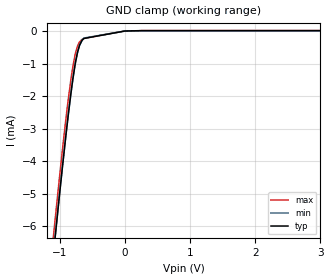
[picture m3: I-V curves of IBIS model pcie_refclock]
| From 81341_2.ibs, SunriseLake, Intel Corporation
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[Model]   pcie_refclock
Model_type   Input
Vinl = 120mV
Vinh = 1000mV
|   typ   min   max
C_comp   600.000fF   500.000fF   700.000fF
[Voltage Range]   1.800V   1.710V   1.890V
[Temperature Range]   60.0   105.0   0.0
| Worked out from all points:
|   GND clamp passes 1 mA (typ) near -0.76 V on its own axis
[GND Clamp]
|   Voltage   I(typ)   I(min)   I(max)
-1.8V     -21.74mA   -21.55mA   -21.76mA
-1.11V    -7.061mA   -7.048mA   -6.513mA
-1.08V    -6.464mA   -6.454mA   -5.917mA
-1.01V    -5.097mA   -5.093mA   -4.558mA
-910mV    -3.236mA   -3.24mA    -2.733mA
-870mV    -2.541mA   -2.549mA   -2.069mA
-800mV    -1.453mA   -1.465mA   -1.079mA
-730mV    -656.1uA   -662.6uA   -463.7uA
-700mV    -445.8uA   -446.4uA   -337.5uA
-630mV    -229.4uA   -216.1uA   -226uA
0V        60.95pA    29.85pA    35.43pA
3.6V      10.65uA    8.798uA    13.22uA
